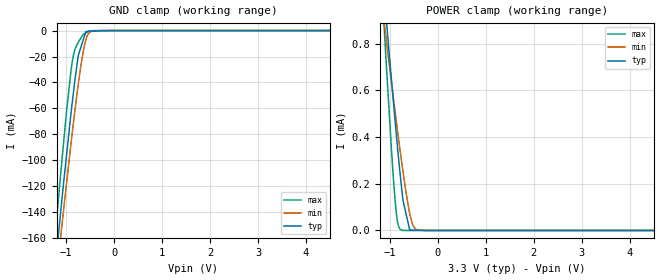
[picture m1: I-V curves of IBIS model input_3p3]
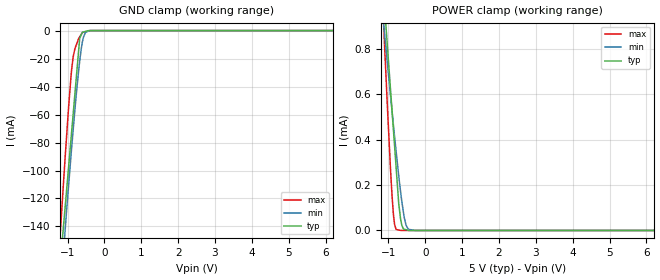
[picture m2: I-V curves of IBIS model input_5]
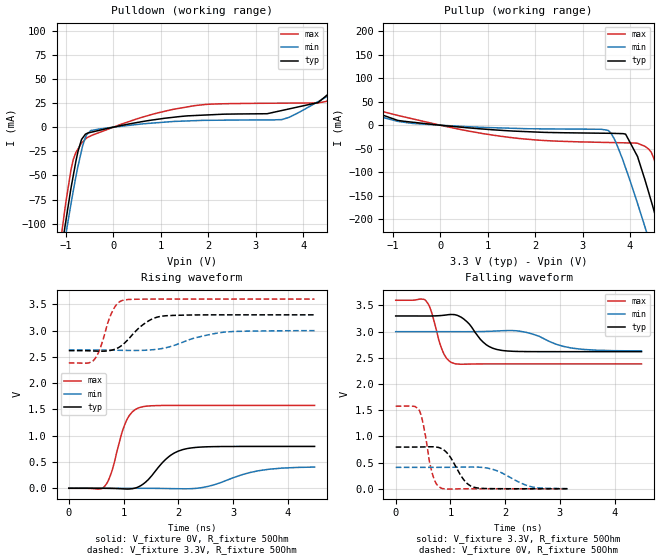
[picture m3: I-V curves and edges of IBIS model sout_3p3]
|Texas Instruments Incorporated
| 16-bit ES-PWM with 7-bit Device Level Brightness Control
| Marketing part#   Digital Voltage Range   Package-type   #pins
| TLC5943PWP   3.0 to 5.5V   HTSSOP   28
| TLC5943PWPG4   3.0 to 5.5V   HTSSOP   28
| TLC5943PWPR   3.0 to 5.5V   HTSSOP   28
| TLC5943PWPRG4   3.0 to 5.5V   HTSSOP   28
| TLC5943RHBR   3.0 to 5.5V   QFN   32
| TLC5943RHBRG4   3.0 to 5.5V   QFN   32
| TLC5943RHBT   3.0 to 5.5V   QFN   32
| TLC5943RHBTG4   3.0 to 5.5V   QFN   32
[IBIS Ver]   3.2
[File name]   tlc5943.ibs
|SIMDE Ver   V2.2 - 201009 - RHL4 - Build 420
[File Rev]   1.0
[Date]   10/19/2010
[Source]
| Texas Instruments Incorporated.
| Analog-eLab Design Center, HPA
| 12500 TI Blvd
| Dallas, TX -75243
| e-mail: elab_ibis@list.ti.com
| -Model generated from simulations in TISPICE
[Notes]   Revision History:
| Rev 1.0: 10/19/2010
| - Initial version of the model
| - Model generated from simulations in TISPICE
| - Model matched to SPICE simulation
| - Model names with a trailing _3p3 contains the model for
|   3.3V [3.0V and 3.6V]. Model names with trailing _5 contains
|   the model for 5.0V [4.5V and 5.5V] operation.
| - C_comp although listed in numerical order of value are
|   obtained from varying PVT conditions. For PVT conditions for
|   each specific value refer the buffer description under
|   respective [Model]. IBIS model user is responsible for using
|   appropriate C_comp to simulate for Signal Integrity.
[Disclaimer]
| This model is designed as an aid for customers of Texas Instruments.
| TI and its licensors and suppliers make no warranties, either expressed
| or implied, with respect to this  model, including the warranties of
| merchantability or fitness for a particular purpose. The model is
| provided solely on an "as is" basis. The entire risk as to its quality
| and performance is with the customer.
[Copyright]
 (C) Copyright 2010 Texas Instruments Incorporated.All rights reserved.
|   TLC5943PWP
[Component]   TLC5943PWP
[Manufacturer]   TI
[Package]   |28 HTSSOP -  PWP package
|   typ   min   max
R_pkg   0.08728   0.05962   0.12307
L_pkg   2.97040nH   2.20454nH   4.21494nH
C_pkg   0.49856pF   0.43432pF   0.62873pF
[Pin]  signal_name   model_name   R_pin   L_pin   C_pin
1   GND   GND   0.04486   3.62079nH  0.71916pF
2   BLANK   INPUT   0.11354   3.80991nH  0.59013pF
3   XLAT   INPUT   0.09593   3.06972nH  0.48021pF
4   SCLK   INPUT   0.08455   2.79380nH  0.47724pF
5   SIN   INPUT   0.07232   2.49922nH  0.45928pF
6   BCSEL   INPUT   0.06409   2.30927nH  0.44108pF
7   OUT0   TERM   0.06002   2.21228nH  0.43432pF
8   OUT1   TERM   0.05962   2.20454nH  0.43472pF
9   OUT2   TERM   0.06529   2.34705nH  0.44709pF
10   OUT3   TERM   0.07503   2.57200nH  0.46399pF
11   OUT4   TERM   0.08868   2.90343nH  0.48671pF
12   OUT5   TERM   0.10604   3.32751nH  0.50100pF
13   OUT6   TERM   0.12307   4.05840nH  0.60900pF
14   OUT7   TERM   0.11419   4.21494nH  0.62873pF
15   OUT8   TERM   0.11417   4.21334nH  0.62830pF
16   OUT9   TERM   0.12301   4.05345nH  0.60885pF
17   OUT10   TERM   0.10604   3.32754nH  0.50099pF
18   OUT11   TERM   0.08868   2.90332nH  0.48675pF
19   OUT12   TERM   0.07503   2.57201nH  0.46398pF
20   OUT13   TERM   0.06529   2.34706nH  0.44709pF
21   OUT14   TERM   0.05962   2.20480nH  0.43475pF
22   OUT15   TERM   0.06002   2.21230nH  0.43623pF
23   XERR   XERR   0.06724   2.38420nH  0.44995pF
24   SOUT   SOUT   0.07793   2.63416nH  0.46952pF
25   GSCLK   INPUT   0.08846   2.88858nH  0.48540pF
26   XTEST   TERM   0.10428   3.27379nH  0.49796pF
27   IREF   TERM   0.11705   3.89366nH  0.59922pF
28   VCC   POWER   0.11359   4.18200nH  0.62746pF
|   TLC5943RHB
[Component]   TLC5943RHB
[Manufacturer]   TI
[Package]   |32 QFN -  RHB package
|   typ   min   max
R_pkg   0.05884   0.04246   0.06962
L_pkg   1.63485nH   1.14802nH   1.96685nH
C_pkg   0.21192pF   0.17925pF   0.23090pF
[Pin]  signal_name   model_name   R_pin   L_pin   C_pin
1   SCLK   INPUT   0.06626   1.86584nH  0.21338pF
2   SIN   INPUT   0.06124   1.70941nH  0.22244pF
3   BCSEL   INPUT   0.05794   1.61050nH  0.21363pF
4   OUT0   TERM   0.05636   1.56351nH  0.21041pF
5   OUT1   TERM   0.05617   1.55791nH  0.21131pF
6   OUT2   TERM   0.05885   1.63760nH  0.21727pF
7   OUT3   TERM   0.06336   1.77282nH  0.22770pF
8   OUT4   TERM   0.06962   1.96685nH  0.22307pF
9   OUT5   TERM   0.06600   1.85715nH  0.21728pF
10   OUT6   TERM   0.05338   1.47321nH  0.20822pF
11   OUT7   TERM   0.04246   1.15060nH  0.17938pF
12   NC   NC   0.00077   0.14191nH  0.10238pF
13   NC   NC   0.00077   0.14192nH  0.10237pF
14   OUT8   TERM   0.04246   1.14802nH  0.17925pF
15   OUT9   TERM   0.05338   1.46673nH  0.20794pF
16   OUT10   TERM   0.06600   1.84826nH  0.21693pF
17   OUT11   TERM   0.06962   1.95574nH  0.22268pF
18   OUT12   TERM   0.06336   1.76101nH  0.22725pF
19   OUT13   TERM   0.05885   1.62500nH  0.21681pF
20   OUT14   TERM   0.05617   1.54501nH  0.21096pF
21   OUT15   TERM   0.05636   1.55062nH  0.21257pF
22   XERR   XERR   0.05996   1.65830nH  0.22250pF
23   SOUT   SOUT   0.06478   1.80372nH  0.23090pF
24   GSCLK   INPUT   0.06890   1.93445nH  0.21898pF
25   XTEST   TERM   0.06431   1.79814nH  0.21112pF
26   IREF   TERM   0.04860   1.32631nH  0.19718pF
27   VCC   POWER   0.04201   1.13559nH  0.17940pF
28   NC   NC   0.00077   0.14192nH  0.10237pF
29   NC   NC   0.00077   0.14191nH  0.10238pF
30   GND   GND   0.01565   0.89846nH  0.23518pF
31   BLANK   INPUT   0.04700   1.28581nH  0.19325pF
32   XLAT   INPUT   0.05852   1.63362nH  0.19742pF
33   thermal_pad   NC   0.00070   0.24678nH  2.29047pF
|   Model Selectors
[Model Selector] INPUT
input_3p3   3.3V digital input
input_5   5.0V digital input
[Model Selector] SOUT
sout_3p3   3.3V digital output
sout_5   5.0V digital output
[Model Selector] XERR
xerr_3p3   3.3V output_open_drain
xerr_5   5.0V output_open_drain
[Model Selector] TERM
term_3-3V   3.3V nominal termination
term_5-0V   5.0V nominal termination
[Model]  term_3-3V
Model_type Terminator
C_comp   1.0e-20F  1.0e-20F  1.0e-20F
|   typ   min   max
[Voltage Range]   3.3V   3.0V   3.6V
[POWER Clamp Reference]   3.3V   3.0V   3.6V
[GND Clamp Reference]   0V   0V   0V
|Ambient Temperature   25   85   -40
|Junction Temperature
[Temperature Range]   65   125   -40
[Model]  term_5-0V
Model_type Terminator
C_comp   1.0e-20F  1.0e-20F  1.0e-20F
|   typ   min   max
[Voltage Range]   5.0V   4.5V   5.5V
[POWER Clamp Reference]   5.0V   4.5V   5.5V
[GND Clamp Reference]   0V   0V   0V
|Ambient Temperature   25   85   -40
|Junction Temperature
[Temperature Range]   65   125   -40
| Models and submodels in the file (8): input_3p3 (Input), input_5 (Input), sout_3p3 (Output), sout_5 (Output), xerr_3p3 (Open_drain), xerr_5 (Open_drain), term_3-3V (Terminator), term_5-0V (Terminator)
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|   input_3p3 Model
[Model]   input_3p3
Model_type   Input
Vinl = 0.99
Vinh = 2.31
|   typ   min   max
|   (nom PVT)   (Fast PVT)   (slow PVT)
|Average
C_comp   1.243e-12   1.241e-12   1.259e-12
| Where nom  PVT is Nominal Process,  3.3V,  65C
|   Fast PVT is Strong Process,   3.6V,  -40C
|   Slow PVT is Weak Process,   3V,  125C
[Model Spec]
Vinl   0.99   0.9   1.08
Vinh   2.31   2.1   2.52
[Voltage Range]   3.3   3   3.6
|Ambient Temperature   25   85   -40
|Junction Temperature
[Temperature Range]   65   125   -40
[Power Clamp Reference]   3.3   3   3.6
[GND Clamp Reference]   0   0   0
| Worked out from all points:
|   GND clamp passes 1 mA (typ) near -0.59 V on its own axis
|   POWER clamp passes 1 mA (typ) near -1.11 V on its own axis
[GND Clamp]
|   Voltage   I(typ)   I(min)   I(max)
-3.3V     -1.048A    -998.8mA   -1.104A
-1.251V   -191.1mA   -207.3mA   -167.9mA
-1.134V   -147.4mA   -166.1mA   -118.7mA
-1.063V   -120.8mA   -141.5mA   -90.41mA
-993.6mV  -96.85mA   -118.5mA   -63.09mA
-867.6mV  -54.12mA   -77.31mA   -22.91mA
-745.8mV  -19.11mA   -41.08mA   -8.901mA
-645mV    -7.363mA   -16.46mA   -3.103mA
-561mV    -532.3uA   -4.08mA    -1.249mA
-483mV    -457.8uA   -588uA     -132.5uA
-285mV    -268.8uA   -2.101uA   -11.61uA
6.6V      0A         0A         0A
[POWER Clamp]
|   Voltage   I(typ)   I(min)   I(max)
-3.3V     6.67mA     4.786mA    9.238mA
-1.181V   1.169mA    999.4uA    1.098mA
-1.084V   928.3uA    831.4uA    742.5uA
-1.023V   779.1uA    728.4uA    535.8uA
-932.4mV  564.9uA    577.1uA    240.1uA
-864mV    407.6uA    464.8uA    71.07uA
-828mV    327.6uA    407uA      23.09uA
-741.6mV  155.7uA    274uA      617nA
-590.7mV  6.052uA    76.61uA    0A
-528mV    757.2nA    27.04uA    0A
-441mV    631.7nA    3.132uA    0A
6.6V      0A         0A         0A
|   input_5 Model
[Model]   input_5
Model_type   Input
Vinl = 1.5
Vinh = 3.5
|   typ   min   max
|   (nom PVT)   (Fast PVT)   (slow PVT)
|Average
C_comp   1.176e-12   1.161e-12   1.273e-12
| Where nom  PVT is Nominal Process,  5V,  65C
|   Fast PVT is Strong Process,   5.5V,  -40C
|   Slow PVT is Weak Process,   4.5V,  125C
[Model Spec]
Vinl   1.5   1.35   1.65
Vinh   3.5   3.15   3.85
[Voltage Range]   5   4.5   5.5
|Ambient Temperature   25   85   -40
|Junction Temperature
[Temperature Range]   65   125   -40
[Power Clamp Reference]   5   4.5   5.5
[GND Clamp Reference]   0   0   0
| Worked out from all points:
|   GND clamp passes 1 mA (typ) near -0.56 V on its own axis
|   POWER clamp passes 1 mA (typ) near -1.11 V on its own axis
[GND Clamp]
|   Voltage   I(typ)   I(min)   I(max)
-5V       -1.796A    -1.692A    -1.901A
-1.21V    -175.5mA   -193.8mA   -150.4mA
-1.14V    -149.2mA   -169.1mA   -121.5mA
-1.067V   -126.9mA   -143.4mA   -91.51mA
-968mV    -96.68mA   -109.9mA   -53.7mA
-885.5mV  -71.48mA   -82.89mA   -27.25mA
-803mV    -46.28mA   -57.7mA    -13.3mA
-670mV    -5.65mA    -21.83mA   -4.497mA
-600mV    -1.266mA   -8.694mA   -1.537mA
-508.5mV  -577.6uA   -1.159mA   -781uA
-396mV    -22.14uA   -51.31uA   -5.121uA
10V       0A         0A         0A
[POWER Clamp]
|   Voltage   I(typ)   I(min)   I(max)
-5V       11.15mA    7.877mA    15.87mA
-1.14V    1.066mA    928.1uA    945.8uA
-1.111V   1.001mA    878.9uA    840.1uA
-1.023V   802.2uA    729.4uA    531.6uA
-902mV    529.3uA    527.5uA    155.9uA
-858mV    430.1uA    455.9uA    60.62uA
-786.5mV  268.8uA    342.1uA    4.269uA
-720mV    118.9uA    241.6uA    2.127uA
-665mV    46.09uA    165uA      354.9nA
-571.5mV  5.217uA    58.41uA    14.57nA
-459mV    944nA      5.127uA    11.73nA
10V       0A         0A         0A
|   sout_3p3 Model
[Model]   sout_3p3
Model_type   Output
Polarity   Non-Inverting
Vmeas = 1.65
Vref = 1.65
Cref = 15pF
Rref = 50
|   typ   min   max
|   (nom PVT)   (Fast PVT)   (slow PVT)
|Average
C_comp   1.904e-12   1.837e-12   1.928e-12
|ON state : BUFFER OUTPUT TURNED HIGH
|C_comp   1.904e-12   1.837e-12   1.928e-12
|OFF state: BUFFER OUTPUT TURNED LOW
|C_comp   1.619e-12   1.594e-12   1.640e-12
| Where nom  PVT is Nominal Process,  3.3V,  65C
|   Fast PVT is Strong Process,   3.6V,  -40C
|   Slow PVT is Weak Process,   3V,  125C
[Voltage Range]   3.3   3   3.6
|Ambient Temperature   25   85   -40
|Junction Temperature
[Temperature Range]   65   125   -40
[Pullup Reference]   3.3   3   3.6
[Pulldown Reference]   0   0   0
[Power Clamp Reference]   3.3   3   3.6
[GND Clamp Reference]   0   0   0
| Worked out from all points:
|   slope of the pulldown table from 0 to 0.495 V, typ, clamps not added: 104 ohm
|   slope of the pullup table from 0 to 0.495 V, typ, clamps not added: 104 ohm
|   falling waveform, V_fixture 3.3V, R_fixture 50Ohm: 20-80 % time 323ps typ, 546ps min, 199ps max; typ from 3.3 V to 2.62 V
|   rising waveform, V_fixture 0V, R_fixture 50Ohm: 20-80 % time 428ps typ, 719ps min, 259ps max; typ from 0 V to 0.796 V
|   rising waveform, V_fixture 3.3V, R_fixture 50Ohm: 20-80 % time 415ps typ, 693ps min, 232ps max; typ from 2.62 V to 3.3 V
|   falling waveform, V_fixture 0V, R_fixture 50Ohm: 20-80 % time 278ps typ, 456ps min, 166ps max; typ from 0.796 V to 0 V
[Pulldown]
|   Voltage   I(typ)   I(min)   I(max)
-3.3V     -989.1mA   -902mA     -1.151A
-1.12V    -136mA     -147.1mA   -120.4mA
-1.049V   -111.7mA   -125.3mA   -94.51mA
-846mV    -49.95mA   -65.73mA   -33.35mA
-673.2mV  -12.79mA   -24.39mA   -16.53mA
-480mV    -5.386mA   -3.605mA   -9.097mA
1.706V    12.01mA    6.701mA    22.24mA
3.555V    17.29mA    7.877mA    24.84mA
4.496V    32.93mA    31.63mA    26.71mA
5.008V    55.43mA    46.6mA     67.09mA
6V        99.11mA    75.65mA    155.8mA
6.6V      125.5mA    93.21mA    209.4mA
[Pullup]
|   Voltage   I(typ)   I(min)   I(max)
-3.3V     110.7mA    76.48mA    210.3mA
-1.181V   20.38mA    15.69mA    28.23mA
1.246V    -10.66mA   -5.705mA   -23.2mA
3.531V    -17.19mA   -10.81mA   -36.83mA
3.66V     -17.44mA   -27.61mA   -37.11mA
3.907V    -19.1mA    -91.25mA   -37.64mA
4.158V    -66.79mA   -166.9mA   -38.53mA
4.316V    -117.2mA   -217.5mA   -45.1mA
4.446V    -161.7mA   -260mA     -57.53mA
4.594V    -214.3mA   -309.6mA   -103.5mA
4.884V    -322.2mA   -408.1mA   -229.6mA
6.6V      -1.009A    -1.018A    -1.045A
[Ramp]
R_load = 50
|   typ   min   max
dV/dt_r   0.477661/4.27044e-10   0.242056/7.12397e-10   0.94593/2.58272e-10
dV/dt_f   0.409108/3.22856e-10   0.220372/5.34895e-10   0.728967/1.98774e-10
[Falling Waveform]
V_fixture = 3.3V
V_fixture_min = 3V
V_fixture_max = 3.6V
R_fixture = 50Ohm
|   Time   V(typ)   V(min)   V(max)
0s        3.3V       3V         3.6V
550ps     3.299V     3V         3.592V
650ps     3.3V       3V         3.389V
870ps     3.313V     3V         2.6V
1.08ns    3.324V     3V         2.39V
1.64ns    2.763V     3.005V     2.385V
1.85ns    2.659V     3.013V     2.385V
2.37ns    2.62V      2.99V      2.385V
3.23ns    2.618V     2.685V     2.385V
4.49ns    2.618V     2.633V     2.385V
[Rising Waveform]
V_fixture = 0V
V_fixture_min = 0V
V_fixture_max = 0V
R_fixture = 50Ohm
|   Time   V(typ)   V(min)   V(max)
0s        217pV      1.746nV    184.6pV
650ps     -603.7uV   274.6uV    32.15mV
780ps     -2.935mV   370.6uV    303.6mV
960ps     -9.626mV   390.7uV    1.022V
1.05ns    -14.26mV   320.4uV    1.28V
1.29ns    36mV       -422.3uV   1.535V
1.84ns    612.3mV    -6.06mV    1.576V
2.14ns    750.5mV    -10.21mV   1.576V
3.48ns    796mV      335.9mV    1.576V
4.49ns    796.1mV    403.4mV    1.577V
[Rising Waveform]
V_fixture = 3.3V
V_fixture_min = 3V
V_fixture_max = 3.6V
R_fixture = 50Ohm
|   Time   V(typ)   V(min)   V(max)
0s        2.618V     2.631V     2.385V
460ps     2.611V     2.631V     2.443V
560ps     2.608V     2.631V     2.628V
800ps     2.632V     2.627V     3.375V
890ps     2.667V     2.626V     3.516V
1ns       2.745V     2.623V     3.581V
1.36ns    3.116V     2.625V     3.598V
1.69ns    3.273V     2.657V     3.6V
2.82ns    3.3V       2.968V     3.6V
4.49ns    3.3V       2.999V     3.6V
[Falling Waveform]
V_fixture = 0V
V_fixture_min = 0V
V_fixture_max = 0V
R_fixture = 50Ohm
|   Time   V(typ)   V(min)   V(max)
0s        796.2mV    408.7mV    1.577V
430ps     797.3mV    408.4mV    1.498V
500ps     798.7mV    408.4mV    1.249V
670ps     802.1mV    408.6mV    287.6mV
840ps     765mV      409.2mV    7.748mV
1.25ns    163.4mV    413.5mV    -171.9uV
1.41ns    34.42mV    415mV      293.7uV
1.79ns    1.968mV    365.8mV    265.7uV
2.49ns    124.3uV    35.35mV    249.1uV
3.14ns    84.1uV     3.16mV     235.2uV
